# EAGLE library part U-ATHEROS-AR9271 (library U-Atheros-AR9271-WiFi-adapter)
Atheros WiFi WLAN device
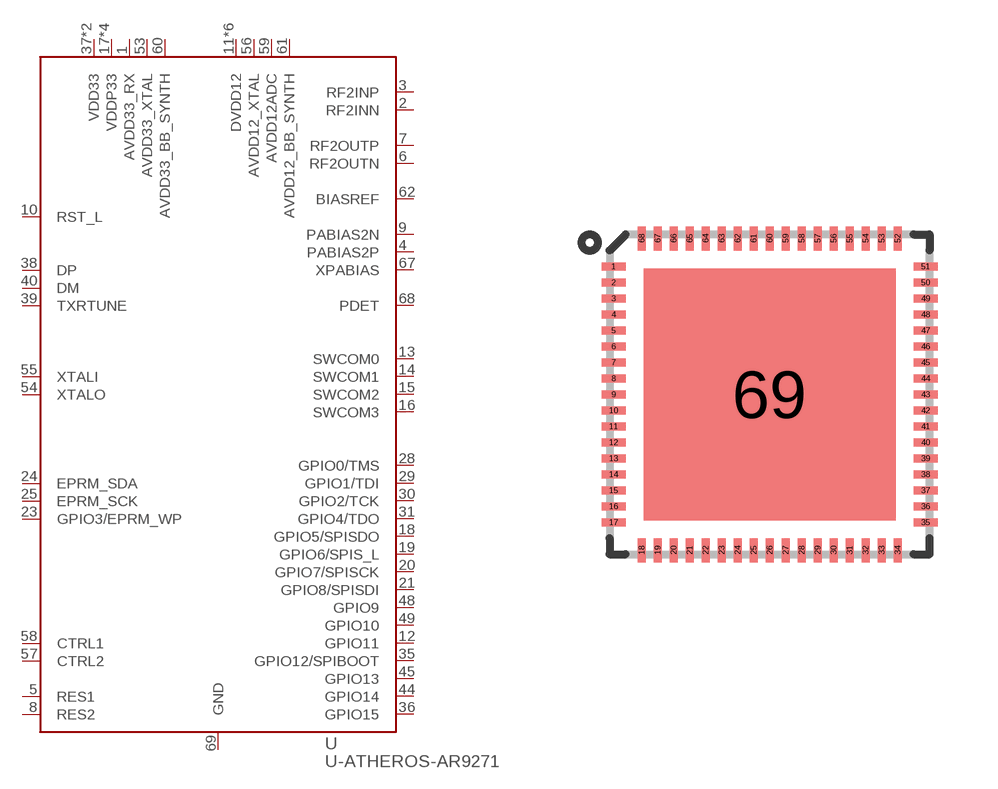
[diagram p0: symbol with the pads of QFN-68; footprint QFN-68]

Designator prefix U

## U-ATHEROS-AR9271  [QFN-68]
1  AVDD33_RX  pwr
2  RF2INN  in
3  RF2INP  in
4  PABIAS2P  in
5  RES1  in
6  RF2OUTN
7  RF2OUTP
8  RES2  in
9  PABIAS2N  in
10  RST_L
11  DVDD12  pwr
12  GPIO11
13  SWCOM0  out
14  SWCOM1  out
15  SWCOM2  out
16  SWCOM3  out
17  VDDP33  pwr
18  GPIO5/SPISDO
19  GPIO6/SPIS_L
20  GPIO7/SPISCK
21  GPIO8/SPISDI
22  DVDD12  pwr
23  GPIO3/EPRM_WP
24  EPRM_SDA
25  EPRM_SCK  out
26  VDDP33  pwr
27  DVDD12  pwr
28  GPIO0/TMS
29  GPIO1/TDI
30  GPIO2/TCK
31  GPIO4/TDO
33  VDDP33  pwr
35  GPIO12/SPIBOOT
36  GPIO15
37  VDD33  pwr
38  DP
39  TXRTUNE
40  DM
41  VDD33  pwr
42  DVDD12  pwr
43  DVDD12  pwr
44  GPIO14
45  GPIO13
46  DVDD12  pwr
47  VDDP33  pwr
48  GPIO9
49  GPIO10
53  AVDD33_XTAL  pwr
54  XTALO  out
55  XTALI  in
56  AVDD12_XTAL  pwr
57  CTRL2
58  CTRL1
59  AVDD12ADC  pwr
60  AVDD33_BB_SYNTH  pwr
61  AVDD12_BB_SYNTH  pwr
62  BIASREF  in
67  XPABIAS  out
68  PDET  in
69  GND  pwr

## Footprint QFN-68 (pad centres in mm)
smd 0.6 x 0.2: 1 -3.9,3.2; 2 -3.9,2.8; 3 -3.9,2.4; 4 -3.9,2; 5 -3.9,1.6; 6 -3.9,1.2; 7 -3.9,0.8; 8 -3.9,0.4; 9 -3.9,0; 10 -3.9,-0.4; 11 -3.9,-0.8; 12 -3.9,-1.2; 13 -3.9,-1.6; 14 -3.9,-2; 15 -3.9,-2.4; 16 -3.9,-2.8; 17 -3.9,-3.2; 35 3.9,-3.2; 36 3.9,-2.8; 37 3.9,-2.4; 38 3.9,-2; 39 3.9,-1.6; 40 3.9,-1.2; 41 3.9,-0.8; 42 3.9,-0.4; 43 3.9,0; 44 3.9,0.4; 45 3.9,0.8; 46 3.9,1.2; 47 3.9,1.6; 48 3.9,2; 49 3.9,2.4; 50 3.9,2.8; 51 3.9,3.2
smd 0.2 x 0.6: 18 -3.2,-3.9; 19 -2.8,-3.9; 20 -2.4,-3.9; 21 -2,-3.9; 22 -1.6,-3.9; 23 -1.2,-3.9; 24 -0.8,-3.9; 25 -0.4,-3.9; 26 0,-3.9; 27 0.4,-3.9; 28 0.8,-3.9; 29 1.2,-3.9; 30 1.6,-3.9; 31 2,-3.9; 32 2.4,-3.9; 33 2.8,-3.9; 34 3.2,-3.9; 52 3.2,3.9; 53 2.8,3.9; 54 2.4,3.9; 55 2,3.9; 56 1.6,3.9; 57 1.2,3.9; 58 0.8,3.9; 59 0.4,3.9; 60 0,3.9; 61 -0.4,3.9; 62 -0.8,3.9; 63 -1.2,3.9; 64 -1.6,3.9; 65 -2,3.9; 66 -2.4,3.9; 67 -2.8,3.9; 68 -3.2,3.9
smd 6.3 x 6.3: 69 0,0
